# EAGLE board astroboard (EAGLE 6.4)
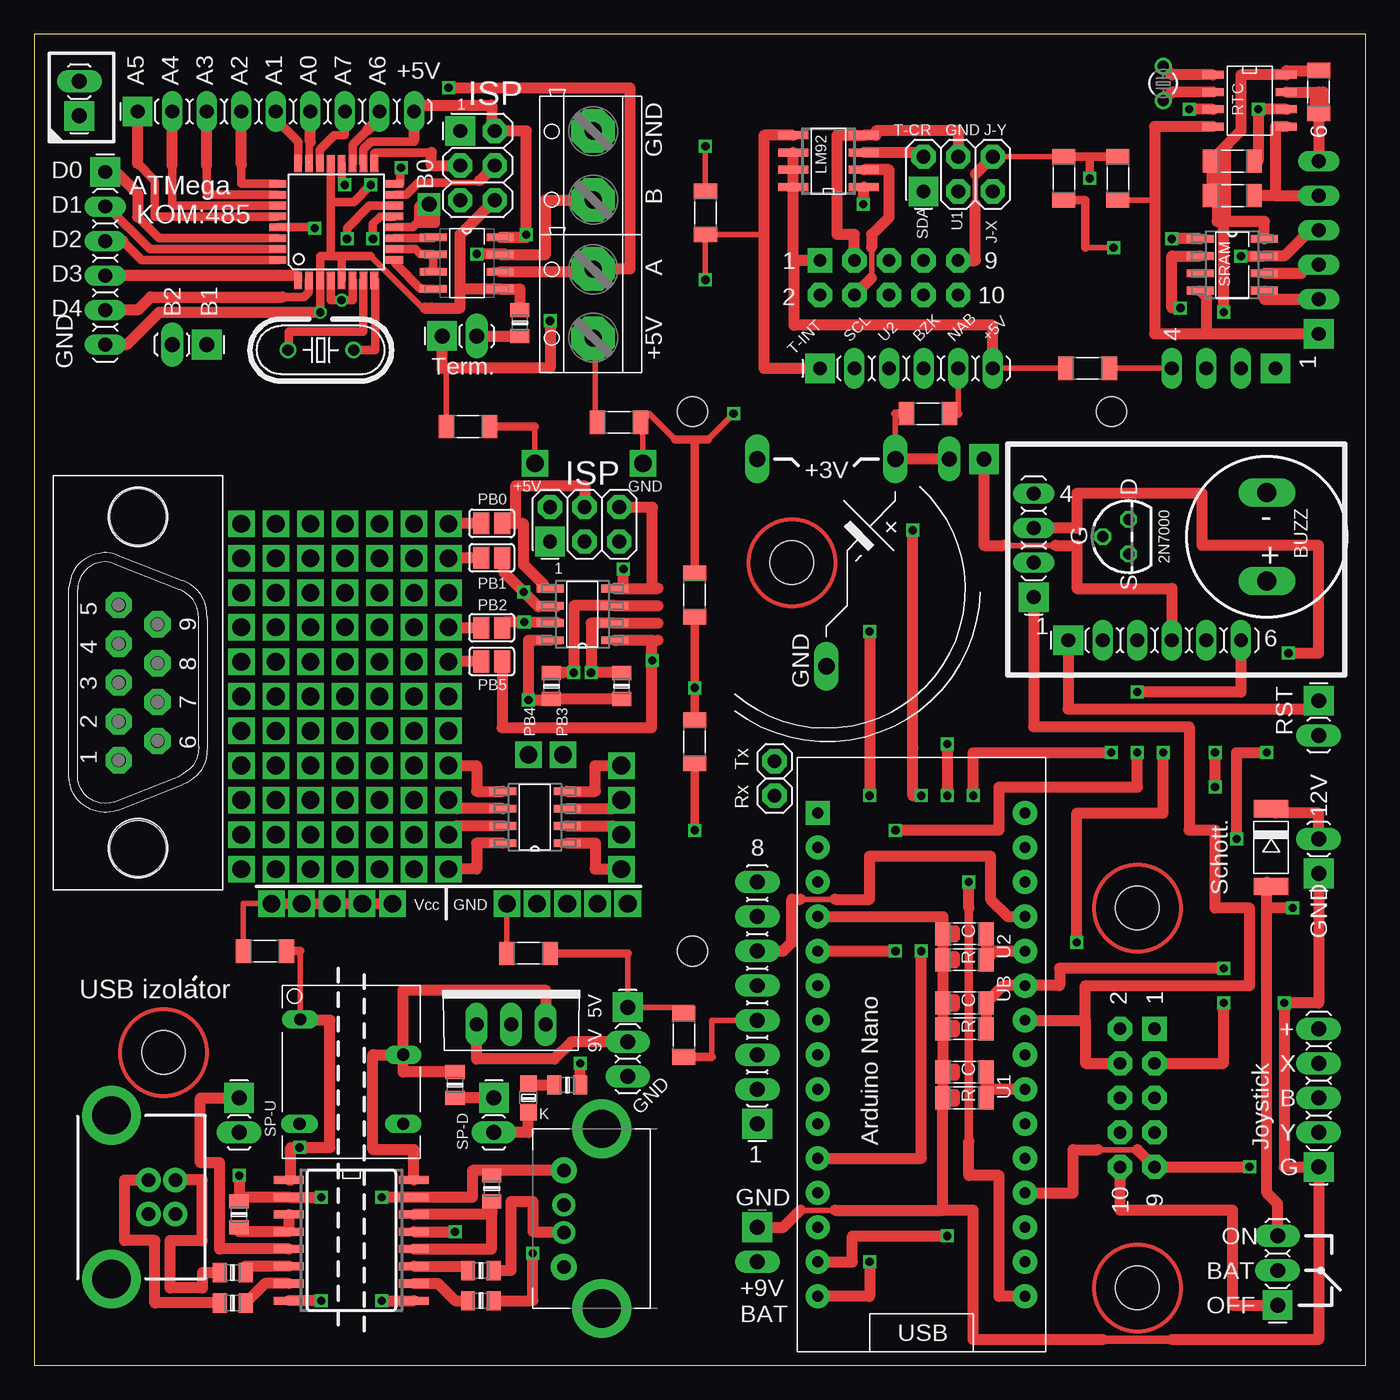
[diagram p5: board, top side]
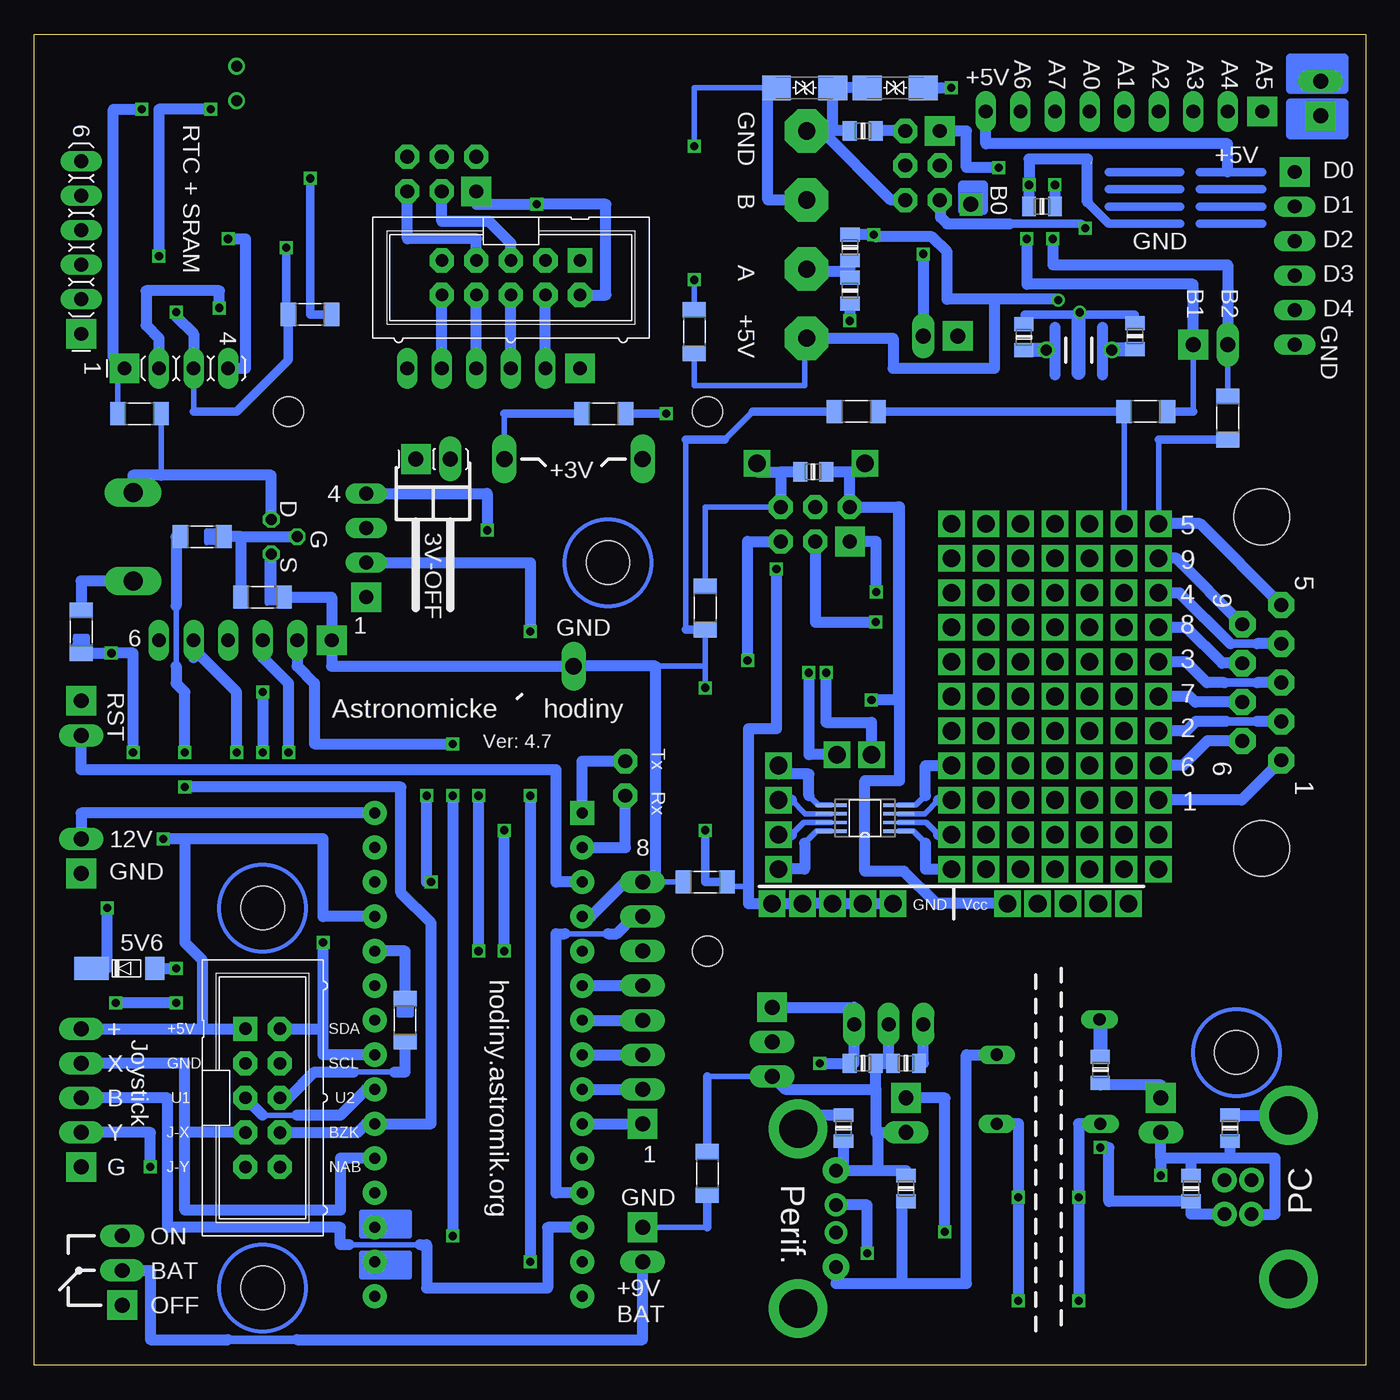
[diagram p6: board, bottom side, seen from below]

Size 97.93 x 97.94 mm. Coordinates in mm from the lower left corner, seen from the top.
Outline: 0,0 97.93,0 97.93,97.94 0,97.94 0,0
Copper layers (1*16): Top 0.0356mm / dielectric 1.5011mm / Bottom 0.0356mm
Design rules "LaenPCBOrder *": minimum track width 6mil, minimum drill 13mil, track to track 6mil, track to pad 6mil, pad to pad 6mil, via to via 6mil, smd to smd 6mil, copper to edge 15mil, drill to drill 6mil, minimum pad ring 7mil, minimum via ring 7mil, stop-mask expansion 3mil, vias tented up to drill 0mil, thermal gap 10mil
Holes 3.2 mm at 81.12,5.71 81.12,33.66 55.72,59.05 9.53,23.02
Holes 2.2 mm at 48.42,70.17 48.42,30.48 79.22,70.17

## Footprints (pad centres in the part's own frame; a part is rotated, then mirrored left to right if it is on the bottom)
BATTERY = drill 1.2 long: + 9.525,-5.08; +@1 9.525,5.08; - -5.715,0
BUZZER-12MM-NS = drill 1.4 long: + 3.25,0; - -3.25,0
1206 = smd 1.143 x 1.702: 1 -1.587,0; 2 1.587,0
0805 = smd 1.016 x 1.422: 1 -0.953,0; 2 0.953,0
CAN9V = drill 1.016 pad 1.93 octagon: 1 -5.715,0; 2 -2.857,0; 3 0,0; 4 2.857,0; 5 5.715,0; 6 -4.286,-2.857; 7 -1.429,-2.857; 8 1.429,-2.857; 9 4.286,-2.857 | hole 4.115: 12.192,-1.429; -12.192,-1.429
SM-1 = smd 1.27 x 2.54: A 2.857,0; K -2.857,0
SOD-80 = smd 1.397 x 1.702: A 1.905,0 | smd 2.54 x 1.702: K -2.731,0
SIM1-0505 = drill 0.9 long: 1 -3.756,3.867; 4 -3.81,-3.81; 5 3.81,-3.81; 7 3.81,1.27
SOIC127P600X175-8N = smd 1.981 x 0.559: 1 -2.362,1.905; 2 -2.362,0.635; 3 -2.362,-0.635; 4 -2.362,-1.905; 5 2.362,-1.905; 6 2.362,-0.635; 7 2.362,0.635; 8 2.362,1.905
TSSOP8 = smd 2.286 x 0.254: 1 -2.489,1.016; 2 -2.489,0.381; 3 -2.489,-0.254; 4 -2.489,-0.889; 5 2.489,-0.889; 6 2.489,-0.254; 7 2.489,0.381; 8 2.489,1.016
TO-220S = drill 1.016 pad 1.6 long: 1 -2.54,0; 2 0,0; 3 2.54,0
1X02 = drill 1.1 pad 2.184 square: 1 -1.27,0 | drill 1.1 long: 2 1.27,0
1X03 = drill 1.1 pad 2.184 square: 1 -2.54,0 | drill 1.1 long: 2 0,0; 3 2.54,0
2X03 = drill 1.016 pad 2.184 square: 1 -2.54,-1.27 | drill 1.016 pad 1.778 octagon: 2 -2.54,1.27; 3 0,-1.27; 4 0,1.27; 5 2.54,-1.27; 6 2.54,1.27
1X06 = drill 1.016 pad 2.184 square: 1 -6.35,0 | drill 1.016 long: 2 -3.81,0; 3 -1.27,0; 4 1.27,0; 5 3.81,0; 6 6.35,0
1X09 = drill 1.016 pad 2.184 square: 1 -10.16,0 | drill 1.016 long: 2 -7.62,0; 3 -5.08,0; 4 -2.54,0; 5 0,0; 6 2.54,0; 7 5.08,0; 8 7.62,0; 9 10.16,0
1X01 = drill 1.3 square: 1 0,0
1X08 = drill 1.1 pad 2.184 square: 1 -8.89,0 | drill 1.1 long: 2 -6.35,0; 3 -3.81,0; 4 -1.27,0; 5 1.27,0; 6 3.81,0; 7 6.35,0; 8 8.89,0
1X05 = drill 1.1 pad 2.184 square: 1 -5.08,0 | drill 1.1 long: 2 -2.54,0; 3 0,0; 4 2.54,0; 5 5.08,0
1X04 = drill 1.016 pad 2.184 square: 1 -3.81,0 | drill 1.016 long: 2 -1.27,0; 3 1.27,0; 4 3.81,0
MLW10G = drill 0.914 pad 1.778 square: 1 -5.08,-1.27 | drill 0.914 pad 1.778 octagon: 2 -5.08,1.27; 3 -2.54,-1.27; 4 -2.54,1.27; 5 0,-1.27; 6 0,1.27; 7 2.54,-1.27; 8 2.54,1.27; 9 5.08,-1.27; 10 5.08,1.27
1X02_OVAL = drill 1.1 pad 2.184 square: 1 -1.27,0 | drill 1.1 long: 2 1.27,0
1X01' = drill 1.016 pad 1.778 octagon: 1 0,0
ARK500/2 = drill 1.27 pad 3.2 octagon: 1 -2.54,0; 2 2.54,0
CHIP-LED0805 = smd 1.2 x 1.2: A 0,-1.05; C 0,1.05
PDIP-32 = drill 0.8 pad 1.778: 3V3 15.24,-35.56; +5V 15.24,-10.16; A0 15.24,-30.48; A1 15.24,-27.94; A2 15.24,-25.4; A3 15.24,-22.86; A4 15.24,-20.32; A5 15.24,-17.78; A6 15.24,-15.24; A7 15.24,-12.7; AREF 15.24,-33.02; D0/RX 0,-5.08; D2 0,-12.7; D3 0,-15.24; D4 0,-17.78; D5 0,-20.32; D6 0,-22.86; D7 0,-25.4; D8 0,-27.94; D9 0,-30.48; D10 0,-33.02; D11 0,-35.56; D12 0,-38.1; D13 15.24,-38.1; GND 0,-10.16; GND1 15.24,-5.08; RESET 0,-7.62; RESET1 15.24,-7.62; VIN 15.24,-2.54 | drill 0.8 pad 1.778 square: D1/TX 0,-2.54
TQFP32-08 = smd 1.27 x 0.559: 1 -4.293,2.8; 2 -4.293,2; 3 -4.293,1.2; 4 -4.293,0.4; 5 -4.293,-0.4; 6 -4.293,-1.2; 7 -4.293,-2; 8 -4.293,-2.8; 17 4.293,-2.8; 18 4.293,-2; 19 4.293,-1.2; 20 4.293,-0.4; 21 4.293,0.4; 22 4.293,1.2; 23 4.293,2; 24 4.293,2.8 | smd 0.559 x 1.27: 9 -2.8,-4.293; 10 -2,-4.293; 11 -1.2,-4.293; 12 -0.4,-4.293; 13 0.4,-4.293; 14 1.2,-4.293; 15 2,-4.293; 16 2.8,-4.293; 25 2.8,4.293; 26 2,4.293; 27 1.2,4.293; 28 0.4,4.293; 29 -0.4,4.293; 30 -1.2,4.293; 31 -2,4.293; 32 -2.8,4.293
TC26V = drill 0.813: 1 -1.27,0; 2 1.27,0
HC49U-V = drill 0.813: 1 -2.413,0; 2 2.413,0
SJ-NC = smd 1.168 x 1.6: 1 -0.762,0; 2 0.762,0
TO-92 = drill 0.813 octagon: 1 -1.27,0; 2 1.27,0; 3 0,1.905
DO214AC+MINIMELF_BIDIR = smd 2.123 x 1.8: P$1 -2.064,0; P$2 2.064,0
SO-8 = smd 0.6 x 1.55: 1 -1.905,-2.69; 2 -0.635,-2.69; 3 0.635,-2.69; 4 1.905,-2.69; 5 1.905,2.71; 6 0.635,2.71; 7 -0.635,2.71; 8 -1.905,2.71
SO08 = smd 0.6 x 2.2: 1 -1.905,-2.6; 2 -0.635,-2.6; 3 0.635,-2.6; 4 1.905,-2.6; 5 1.905,2.6; 6 0.635,2.6; 7 -0.635,2.6; 8 -1.905,2.6
SO16W = smd 0.6 x 2.2: 1 -4.445,-4.6; 2 -3.175,-4.6; 3 -1.905,-4.6; 4 -0.635,-4.6; 5 0.635,-4.6; 6 1.905,-4.6; 7 3.175,-4.6; 8 4.445,-4.6; 9 4.445,4.6; 10 3.175,4.6; 11 1.905,4.6; 12 0.635,4.6; 13 -0.635,4.6; 14 -1.905,4.6; 15 -3.175,4.6; 16 -4.445,4.6
SOIC127P600X175-8N' = smd 1.981 x 0.559: 1 -2.464,1.905; 2 -2.464,0.635; 3 -2.464,-0.635; 4 -2.464,-1.905; 5 2.464,-1.905; 6 2.464,-0.635; 7 2.464,0.635; 8 2.464,1.905
USB-B-PTH = drill 1 pad 1.778: D+ 0,1.25; D- 1.981,1.25; GND 0,-1.25; VBUS 1.981,-1.25 | drill 2.8 pad 4.318: P$2 -2.718,6.02; SHIELD -2.718,-6.02
USB-A-H = drill 1 pad 1.676: D+ 2.794,-1.016; D- 2.794,1.016 | drill 1 pad 1.93: GND 2.794,-3.556; VBUS 2.794,3.556 | drill 2.8 pad 4.318: SHIELD@1 0,-6.604; SHIELD@2 0,6.604

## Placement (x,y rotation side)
BAT3V  3V  [BATTERY]  58.26,57.15 90 top
BUZZ  LD-BZEN1205  [BUZZER-12MM-NS]  90.65,60.96 270 top
C1  100n  [1206]  68.42,24.77 0 top
C2  100n  [1206]  68.42,29.84 0 top
C3  100n  [1206]  68.42,19.68 0 top
C4  100n  [0805]  12.86,13.02 90 bottom
C5  100n  [0805]  15.08,11.11 90 top
C6  100n  [0805]  10,17.46 270 bottom
C7  100n  [0805]  33.81,13.02 90 bottom
C8  100n  [0805]  33.66,13.02 90 top
C9  100n  [0805]  38.42,17.46 90 bottom
C10  100n  [0805]  36.99,22.23 0 bottom
C11  100n  [0805]  33.81,22.23 180 bottom
C12  1u  [0805]  23.81,85.25 180 bottom
C13  18p  [0805]  16.98,75.71 90 bottom
C14  18p  [0805]  25.15,75.63 90 bottom
C15  1uF  [0805]  36.99,90.81 0 bottom
C16  1uF  [0805]  40.64,65.72 180 bottom
CAN1  CAN_9V  [CAN9V]  6.22,50.23 90 top
D1  SK110  [SM-1]  90.96,38.1 270 top
D2  5V6  [SOD-80]  90.96,29.21 0 bottom
DC-DC1  [SIM1-0505]  23.34,21.59 0 top
EMPTY1  SOIC-NIC  [SOIC127P600X175-8N]  36.83,40.32 180 top
EMPTY2  TSSOP-NIC  [TSSOP8]  36.83,40.32 180 bottom
IO1  7805  [TO-220S]  35.08,25.08 0 top
JP1  [1X02]  15.08,18.41 270 top
JP2  [1X02]  33.81,18.41 270 top
JP3  [1X03]  43.66,23.81 270 top
JP4  [1X02]  31.27,75.72 0 top
JP5  [2X03]  32.61,88.26 270 top
JP6  [1X06]  5.24,81.44 270 top
JP7  [1X02]  11.43,75.09 180 top
JP8  [1X09]  17.78,92.23 0 top
JP9  [1X02]  3.33,93.19 90 top
JP10  [2X03]  40.48,61.88 0 top
JP11  [1X01]  30.48,39.05 0 top
JP12  [1X01]  30.48,41.59 0 top
JP13  [1X01]  30.48,44.13 0 top
JP14  [1X01]  43.18,36.51 180 top
JP15  [1X01]  43.18,39.05 180 top
JP16  [1X01]  43.18,41.59 180 top
JP17  [1X01]  43.18,44.13 180 top
JP18  [1X01]  15.24,41.59 0 top
JP19  [1X01]  15.24,46.67 180 top
JP20  [1X01]  15.24,51.75 180 top
JP21  [1X01]  15.24,56.83 180 top
JP22  [1X01]  15.24,61.91 180 top
JP23  [1X01]  15.24,44.13 180 top
JP24  [1X01]  15.24,49.21 180 top
JP25  [1X01]  15.24,54.29 180 top
JP26  [1X01]  15.24,59.37 180 top
JP27  [1X01]  30.48,61.91 90 top
JP28  [1X01]  30.48,59.37 90 top
JP29  [1X01]  30.48,54.29 90 top
JP30  [1X01]  30.48,51.75 90 top
JP31  [1X01]  38.89,44.93 90 top
JP32  [1X01]  36.35,44.93 90 top
JP33  [1X01]  22.86,39.05 0 top
JP34  [1X01]  17.78,61.91 0 top
JP35  [1X01]  20.32,61.91 0 top
JP36  [1X01]  22.86,61.91 0 top
JP37  [1X01]  17.78,59.37 0 top
JP38  [1X01]  25.4,61.91 0 top
JP39  [1X01]  27.94,61.91 0 top
JP40  [1X01]  20.32,59.37 0 top
JP41  [1X01]  25.4,59.37 0 top
JP42  [1X01]  22.86,59.37 0 top
JP43  [1X01]  17.78,56.83 0 top
JP44  [1X01]  27.94,59.37 0 top
JP45  [1X01]  20.32,56.83 0 top
JP46  [1X01]  22.86,56.83 0 top
JP47  [1X01]  25.4,56.83 0 top
JP48  [1X01]  27.94,56.83 0 top
JP49  [1X01]  17.78,54.29 0 top
JP50  [1X01]  30.48,56.83 0 top
JP51  [1X01]  25.4,41.59 0 top
JP52  [1X01]  22.86,51.75 0 top
JP53  [1X01]  20.32,54.29 0 top
JP54  [1X01]  22.86,46.67 0 top
JP55  [1X01]  27.94,49.21 0 top
JP56  [1X01]  25.4,54.29 0 top
JP57  [1X01]  20.32,46.67 0 top
JP58  [1X01]  30.48,49.21 0 top
JP59  [1X01]  27.94,54.29 0 top
JP60  [1X01]  22.86,54.29 0 top
JP61  [1X01]  17.78,46.67 0 top
JP62  [1X01]  30.48,46.67 0 top
JP63  [1X01]  25.4,51.75 0 top
JP64  [1X01]  17.78,51.75 0 top
JP65  [1X01]  17.78,44.13 0 top
JP66  [1X01]  27.94,46.67 0 top
JP67  [1X01]  20.32,49.21 0 top
JP68  [1X01]  17.78,49.21 0 top
JP69  [1X01]  25.4,39.05 0 top
JP70  [1X01]  25.4,46.67 0 top
JP71  [1X01]  22.86,49.21 0 top
JP72  [1X01]  20.32,51.75 0 top
JP73  [1X01]  20.32,44.13 0 top
JP74  [1X01]  25.4,44.13 0 top
JP75  [1X01]  25.4,49.21 0 top
JP76  [1X01]  27.94,51.75 0 top
JP77  [1X01]  22.86,41.59 0 top
JP78  [1X01]  20.32,41.59 0 top
JP79  [1X01]  17.78,41.59 0 top
JP80  [1X01]  22.86,44.13 0 top
JP81  [1X01]  15.24,36.51 0 top
JP82  [1X01]  20.32,39.05 0 top
JP83  [1X01]  17.78,36.51 0 top
JP84  [1X01]  17.78,39.05 0 top
JP85  [1X01]  20.32,36.51 0 top
JP86  [1X01]  15.24,39.05 0 top
JP87  [1X01]  25.4,36.51 0 top
JP88  [1X01]  22.86,36.51 0 top
JP89  [1X01]  27.94,44.13 0 top
JP90  [1X01]  27.94,41.59 0 top
JP91  [1X01]  27.94,39.05 0 top
JP92  [1X01]  27.94,36.51 0 top
JP93  [1X01]  34.77,33.97 0 top
JP94  [1X01]  44.77,66.36 0 top
JP95  [1X01]  36.83,66.36 0 top
JP97  [1X01]  36.99,33.97 0 top
JP98  [1X01]  39.21,33.97 0 top
JP99  [1X01]  41.43,33.97 0 top
JP100  [1X01]  43.66,33.97 0 top
JP101  [1X01]  19.68,33.97 0 top
JP103  [1X01]  21.91,33.97 0 top
JP104  [1X01]  17.46,33.97 0 top
JP105  [1X01]  26.35,33.97 0 top
JP106  [1X01]  24.13,33.97 0 top
JP108  [1X01]  30.48,36.51 0 top
K1  [1X08]  53.18,26.67 90 top
K2  [1X05]  94.46,19.68 90 top
K3A  [1X04]  73.5,60.33 90 top
K3B  [1X04]  87.47,73.34 180 top
K4A  [1X06]  82.39,53.34 0 top
K4B  [1X06]  94.46,82.23 90 top
K5  MLW10  [MLW10G]  81.12,19.68 270 bottom
K6  [1X02]  94.46,37.47 90 top
K7  [1X02_OVAL]  53.18,8.89 270 top
K8  [1X03]  91.44,6.99 90 top
K9  [1X02]  94.46,47.62 270 top
K10  [1X01']  54.45,44.45 0 top
K11  [1X01']  54.45,41.91 0 top
K12  [1X02]  68.58,66.67 0 bottom
K13  MLW10  [MLW10G]  62.87,80.01 180 bottom
K14  [2X03]  67.94,87.63 0 top
K15  [1X06]  64.14,73.34 0 top
K16A  ARK500/2  [ARK500/2]  41.12,78.11 90 top
K16B  ARK500/2  [ARK500/2]  41.12,88.27 90 top
LED1  [CHIP-LED0805]  36.35,19.68 180 top
MCU1  ARDUINONANO  [PDIP-32]  57.63,43.18 0 top
MCU2  ATTINY__  [SOIC127P600X175-8N]  40.32,55.24 180 top
MCU3  ATmega328  [TQFP32-08]  22.22,84.11 90 top
Q1  32768Hz  [TC26V]  83.03,94.3 90 top
Q2  16MHz  [HC49U-V]  21.09,74.69 180 top
R1  4k7  [1206]  85.57,60.96 0 bottom
R2  18k  [1206]  81.12,56.52 180 bottom
R3  330R  [1206]  94.46,53.98 90 bottom
R4  3k3  [1206]  94.46,93.66 90 top
R5  3k3  [1206]  88.11,88.58 180 top
R6  3k3  [1206]  88.11,86.04 180 top
R7  10k  [1206]  68.42,26.67 0 top
R8  1k  [1206]  75.72,87.31 90 top
R8-A  0R  [1206]  70.64,25.4 270 bottom
R8-B  10k  [1206]  68.42,31.75 0 top
R9  10k  [1206]  68.42,21.59 0 top
R10  24R 1%  [0805]  14.61,6.83 0 top
R11  24R 1%  [0805]  14.61,4.6 0 top
R12  47k  [0805]  19.53,21.75 90 bottom
R13  24R 1%  [0805]  32.86,6.99 0 top
R14  24R 1%  [0805]  32.86,4.76 0 top
R15  47k  [0805]  30.96,20.64 90 top
R16  1k  [0805]  39.21,20.64 0 top
R17  47k  [0805]  35.72,76.68 90 top
R18  47k  [0805]  37.94,82.23 270 bottom
R19  120R  [0805]  37.94,79.06 90 bottom
R20  47k  [0805]  43.21,49.97 270 top
R21  47k  [0805]  38.04,49.97 270 top
R22  1k  [1206]  79.69,87.31 270 top
R23  1k  [1206]  90.17,70.01 180 bottom
R24  1k  [1206]  65.72,70.01 0 top
R25  1k  [1206]  77.47,73.34 180 top
R26  1k  [1206]  49.37,84.77 90 top
R27  1k  [1206]  48.58,35.56 0 bottom
R28  1k  [1206]  48.58,55.72 90 bottom
R29  1k  [1206]  48.58,45.88 270 top
R30  1k  [1206]  10.16,69.69 270 bottom
R31  1k  [1206]  49.37,76.04 270 bottom
R32  1k  [1206]  16.19,70.17 180 bottom
R33  1k  [1206]  77.63,77.31 180 bottom
R34  1k  [1206]  31.91,69.06 0 top
R35  1k  [1206]  43.02,69.37 180 top
R36  1k  [1206]  47.78,24.29 270 top
R37  1k  [1206]  48.42,14.13 270 bottom
R38  1k  [1206]  16.99,30.48 0 top
R39  1k  [1206]  36.35,30.32 0 top
R40  1k  [1206]  37.47,70.17 0 bottom
R41  1k  [1206]  48.58,56.67 270 top
R42  1k  [1206]  56.04,70.01 180 bottom
SJ-B0  SOLDERJUMPERNC  [SJ-NC]  33.66,61.94 180 top
SJ-B1  SOLDERJUMPERNC  [SJ-NC]  33.66,59.4 180 top
SJ-B2  SOLDERJUMPERNC  [SJ-NC]  33.66,54.26 180 top
SJ-B5  SOLDERJUMPERNC  [SJ-NC]  33.66,51.78 180 top
T1  2N7000  [TO-92]  80.49,60.96 90 top
TR1  6V8  [DO214AC+MINIMELF_BIDIR]  41.27,93.98 180 bottom
TR2  6V8  [DO214AC+MINIMELF_BIDIR]  34.61,93.98 0 bottom
U1  23LCV512-I/SN  [SOIC127P600X175-8N]  88.11,80.96 0 top
U2  RTC-M41T81M6F  [SO-8]  89.38,93.03 270 top
U3  LM92  [SO08]  58.42,88.58 90 top
U4  ADuM4160  [SO16W]  23.34,9.21 270 top
U5  ADM485ARZ  [SOIC127P600X175-8N']  31.83,81.08 0 top
X1  USB B  [USB-B-PTH]  8.41,12.38 0 top
X2  USB A  [USB-A-H]  41.75,10.79 180 top

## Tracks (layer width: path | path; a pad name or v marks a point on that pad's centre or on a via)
+3V(BAT)
  Top 0.406: 71.28,60.33 75.09,60.33
  Top 0.813: K4A.4 83.66,57.15 76.68,57.15 76.68,60.33 75.09,60.33 | 71.28,60.33 69.85,60.33 K12.1
+3V(BAT)-ED  (via drill 0.6)
  Top 0.813: U2.3 v84.93,92.39 | v88.74,81.6 U1.7 91.92,81.6 93.82,83.5 K4B.4
  Bottom 0.813: v84.93,92.39 88.74,92.39 v88.74,81.6
+5V  (via drill 0.6)
  Top 0.406: 56.36,34.29 58.9,34.29
  Top 0.813: K1.6 55.09,30.48 55.72,31.11 55.72,34.29 56.36,34.29 | MCU1.+5V 71.6,33.02 70.33,34.29 70.33,37.47 61.44,37.47 61.44,34.29 58.9,34.29 | v92.23,52.39 R3.1 94.46,60.33 85.88,60.33 85.88,64.14 76.68,64.14 76.68,61.59 K3A.3 | v88.42,38.73 88.42,45.09 v90.65,45.09
  Bottom 0.305: 94.93,52.86 94.93,53.18 | 94.93,53.5 94.93,53.66 93.98,53.66 93.98,53.5 | 94.93,53.34 94.93,53.18 | 94.93,53.18 94.14,53.18 | 93.98,53.5 93.98,53.34 | 93.98,53.34 93.98,53.02 | 93.98,53.34 94.93,53.34 | 94.93,53.34 94.93,53.5 | 94.93,53.5 93.98,53.5
  Bottom 0.406: 93.82,52.86 94.46,52.86 | 94.46,52.86 94.93,52.86 95.09,52.86 | R3.1 94.46,52.86
  Bottom 0.813: K2.5 85.57,24.77 | 85.57,24.77 K5.1 | MCU1.+5V 76.68,33.02 76.68,38.73 86.84,38.73 | 86.84,38.73 86.84,31.11 85.57,29.84 85.57,24.77 | 86.84,38.73 v88.42,38.73 | v90.65,45.09 90.65,52.39 v92.23,52.39 R3.1
+5V-ED  (via drill 0.6)
  Top 0.406: 87.47,84.14 87.47,84.45 | v79.38,82.23 77.31,82.23
  Top 0.61: U2.8 92.09,95.25 | R6.2 R5.2 87,89.06 | R8.1 77.31,85.72 77.31,82.23
  Top 0.813: 92.09,95.25 R4.2 | U2.8 88.74,94.93 88.74,90.81 87,89.06 87,84.14 87.47,84.14 | U1.8 90.47,84.14 87.47,84.14 | v87.47,77.47 87.47,84.14
  Top 1.016: 87.47,89.38 87.47,84.45
  Bottom 0.406: R33.2 79.38,77.31 79.38,73.66 | 86.2,70.17 K3B.3
  Bottom 0.61: 79.38,77.31 v79.38,82.23 | 86.2,70.17 83.03,70.17 79.22,73.98 R33.2
  Bottom 0.813: v87.47,77.47 87.47,77.15 86.2,75.88 K3B.3
+5V-TP
  Top 0.406: R25.2 K15.6
  Top 0.813: K13.1 55.88,81.28 | 55.88,81.28 55.82,81.28 U3.8 U3.7 U3.6 | K15.6 70.48,76.52 55.88,76.52 55.88,81.28
ARDU/3V3
  Bottom 0.406: MCU1.3V3 70.33,7.62 | 70.33,7.62 70.33,7.3 | 70.33,7.3 70.33,6.51 73.82,6.51 73.82,8.26 70.33,8.26 70.33,7.62 | 70.33,7.3 70.64,7.3 | 70.64,6.99 70.64,6.67 73.5,6.67 73.5,7.3 70.64,7.3 | 70.64,7.3 70.64,7.94 73.18,7.94 73.18,7.62 | 70.64,7.3 70.64,6.99 | 70.64,6.99 73.34,6.99 73.34,7.46 72.55,7.46
  Bottom 0.61: 73.18,7.62 73.18,7.3
ARDU/A0  (via drill 0.6)
  Top 0.406: 78.23,15.88 81.12,15.88
  Top 0.813: v89.38,14.61 K5.9 81.12,15.88 | MCU1.A0 76.4,12.7 76.4,15.88 78.23,15.88
  Bottom 0.813: v89.38,14.61 89.38,17.14 K2.2
ARDU/A0-TP  (via drill 0.6)
  Top 0.406: 69.22,85.41 69.22,87.63 | K14.6 R8.2
  Top 0.61: R8.2 77.63,88.9 | 77.63,88.9 R22.1 | v77.63,87.31 77.63,88.9
  Top 0.813: K13.9 69.22,81.28 69.22,85.41 | 69.22,87.63 K14.6
  Bottom 0.61: R33.1 77.63,77.31 v77.63,87.31
ARDU/A1
  Bottom 0.813: MCU1.A1 75.41,15.24 75.41,11.43 86.84,11.43 86.84,17.14 | 86.84,17.14 86.84,22.23 K2.4 | K5.7 86.84,17.14
ARDU/A1-TP
  Bottom 0.813: K13.7 65.41,82.87 70.48,82.87 K14.5
ARDU/A2  (via drill 0.6)
  Top 0.813: v86.84,42.55 v86.84,45.09
  Bottom 0.406: 87.47,55.88 87.47,51.44
  Bottom 0.813: v86.84,42.55 70.96,42.55 70.96,34.77 68.74,32.54 68.74,17.78 MCU1.A2 73.5,17.78 74.14,17.14 K5.8 | v86.84,45.09 86.84,49.53 87.47,50.16 87.47,51.44 | R1.1 87.47,60.96 87.47,55.88
ARDU/A2-TP
  Bottom 0.813: K15.4 K13.8
ARDU/A3
  Top 0.61: C3.2 70.01,20.32
  Top 0.813: R9.2 70.01,20.32 MCU1.A3
  Bottom 0.406: 78.58,18.41 81.12,18.41
  Bottom 0.813: K5.5 81.12,18.41 | MCU1.A3 73.5,20.32 75.41,18.41 78.58,18.41
ARDU/A3-TP
  Bottom 0.813: K13.5 62.87,82.55 64.45,84.14 67.94,84.14 K14.3
ARDU/A4  (via drill 0.6)
  Top 0.813: v76.68,31.11 76.68,40.64 83.03,40.64 v83.03,45.09
  Bottom 0.813: MCU1.A4 76.68,22.86 76.68,24.77 | K5.2 76.68,24.77 | 76.68,24.77 v76.68,31.11 | v83.03,45.09 83.03,49.53 86.2,52.7 | 86.2,52.07 86.2,52.7 | 86.2,52.7 K4A.5
ARDU/A4-ED
  Top 0.813: U2.5 91.28,91.12 91.28,86.04 | 91.28,86.04 R6.1 | 91.28,86.04 K4B.5
ARDU/A4-TP  (via drill 0.6)
  Top 0.406: v60.96,85.41 61.02,85.41
  Top 0.813: 61.02,85.41 U3.1
  Bottom 0.813: K13.2 55.88,78.74 55.88,85.41 v60.96,85.41 65.41,85.41 K14.1
ARDU/A5
  Top 0.813: MCU1.A5 77.31,25.4 | 77.31,25.4 77.31,22.23 K5.4 | K3A.1 73.5,46.99 84.93,46.99 84.93,39.37 86.84,39.37 86.84,33.66 89.38,33.66 89.38,27.94 77.31,27.94 77.31,25.4
ARDU/A5-ED  (via drill 0.6)
  Top 0.61: 90.01,88.58 R5.1
  Top 0.813: U2.6 v90.01,92.39 90.01,88.58
  Bottom 0.406: K3B.1 91.76,73.34 R23.2
  Bottom 0.813: K3B.1 92.09,74.15 U2.6 v90.01,92.39
ARDU/A5-TP
  Top 0.406: 61.59,82.23 61.59,80.01
  Top 0.813: K13.4 61.59,80.01 | U3.2 62.87,87.95 62.87,84.45 61.59,83.19 61.59,82.23
  Bottom 0.813: K15.2 K13.4
ARDU/A6  (via drill 0.6)
  Top 0.813: C1.2 R7.2 71.28,27.94 MCU1.A6 75.41,27.94 75.41,29.21 v87.47,29.21
  Bottom 0.813: D2.A v87.47,29.21
ARDU/A7
  Top 0.813: R8-B.2 C2.2 70.64,30.48 MCU1.A7
  Bottom 0.305: 70.17,26.51 70.17,25.72 71.12,25.72 71.12,26.51 70.33,26.51 70.33,25.88 70.96,25.88 70.96,26.35 70.48,26.35 70.48,26.04 | 70.8,26.04 70.8,26.19
  Bottom 0.406: 70.48,26.04 70.8,26.04 | 70.33,26.51 70.64,26.51 R8-A.1
  Bottom 0.813: R8-A.1 70.64,30.48 MCU1.A7
ARDU/A7-TP
  Bottom 0.813: K15.3 K13.6
ARDU/AREF
  Bottom 0.406: MCU1.AREF 70.33,10.16 | 70.33,10.16 70.33,9.84 | 70.33,9.84 70.33,9.53 73.82,9.53 73.82,11.27 70.33,11.27 70.33,10.64 | 70.33,10.16 70.33,10.48 70.33,10.64 | 70.33,9.84 73.5,9.84 73.5,10 | 73.5,10.64 73.5,10.95 70.64,10.95 70.64,10.48 73.18,10.48 73.18,10 73.5,10 | 73.5,10 73.5,10.64 | 73.5,10.64 70.33,10.64
ARDU/D0
  Bottom 0.813: MCU1.D0/RX 54.45,38.1 K11.1
ARDU/D1
  Bottom 0.813: MCU1.D1/TX 57.63,44.45 K10.1
ARDU/D2  (via drill 0.6)
  Top 0.813: MCU1.D2 v63.34,30.48 | K4A.6 88.74,49.53 v81.12,49.53 | v63.34,39.37 70.96,39.37 70.96,42.55 81.12,42.55 v81.12,45.09
  Bottom 0.813: v81.12,49.53 v81.12,45.09 | v63.34,30.48 v63.34,39.37
ARDU/D2-ED
  Top 0.406: 93.98,92.71 94.93,92.71 94.93,93.66 | 93.98,93.03 94.93,93.03 | 93.98,93.03 93.98,93.5 | 94.93,93.66 94.93,93.82 | 94.77,93.66 94.93,93.66 | 93.98,92.55 93.98,92.71 | 93.98,93.03 93.98,92.87 93.98,92.71
  Top 0.813: U2.7 94.46,93.66 | 94.46,93.66 R4.1 K4B.6 | 94.46,93.66 94.77,93.66 94.77,92.55
ARDU/D3
  Bottom 0.813: MCU1.D3 K1.5
ARDU/D4
  Top 0.406: 49.85,22.7 49.85,25.4 K1.4
  Top 0.61: R36.2 49.85,22.7
  Bottom 0.813: MCU1.D4 K1.4
ARDU/D5
  Bottom 0.813: MCU1.D5 K1.3
ARDU/D6
  Bottom 0.813: MCU1.D6 K1.2
ARDU/D7
  Bottom 0.813: MCU1.D7 K1.1
ARDU/D8  (via drill 0.6)
  Top 0.813: MCU1.D8 65.25,15.24 v65.25,30.48 | v65.25,41.91 64.61,41.91 64.61,45.4 v64.61,61.44
  Bottom 0.813: v65.25,30.48 v65.25,41.91 | K3A.4 64.61,64.14 v64.61,61.44
ARDU/D8-ED  (via drill 0.6)
  Top 0.406: R25.1 K3B.4
  Top 0.813: U1.1 v83.66,82.87
  Bottom 0.813: v83.66,82.87 82.39,82.87 82.39,73.34 K3B.4
ARDU/D9
  Bottom 0.406: 58.9,31.75 55.72,31.75
  Bottom 0.813: MCU1.D9 59.53,12.7 59.53,31.75 58.9,31.75 | 55.72,31.75 55.09,31.75 53.82,33.02 K1.7
ARDU/D10
  Bottom 0.406: 69.53,8.89 74.77,8.89
  Bottom 0.813: K2.3 88.11,19.68 88.11,10.16 75.41,10.16 75.41,8.89 74.77,8.89 | MCU1.D10 60.17,10.16 60.17,5.71 69.06,5.71 69.06,8.89 69.53,8.89
ARDU/D11  (via drill 0.6)
  Top 0.813: v67.15,45.72 v67.15,41.91 | MCU1.D11 60.17,7.62 60.17,9.53 v67.15,9.53
  Bottom 0.813: K4A.2 78.58,51.44 77.31,50.16 77.31,45.72 v67.15,45.72 | v67.15,41.91 v67.15,9.53
ARDU/D11-ED
  Top 0.813: U1.5 90.47,78.42 K4B.2
ARDU/D12  (via drill 0.6)
  Top 0.813: v61.44,53.98 v61.44,41.91 | v61.44,7.62 61.44,5.08 MCU1.D12
  Bottom 0.813: K3A.2 61.44,59.05 v61.44,53.98 | v61.44,41.91 v61.44,7.62
ARDU/D12-ED  (via drill 0.6)
  Top 0.813: v84.3,77.79 83.66,77.79 83.66,81.6 U1.2
  Bottom 0.813: v84.3,77.79 84.3,79.06 89.69,79.06 89.69,76.52 88.74,75.56 K3B.2
ARDU/D13  (via drill 0.6)
  Top 0.61: 68.74,16.51 68.74,33.66
  Top 0.813: MCU1.D13 70.96,5.08 70.96,13.97 68.74,13.97 68.74,16.51 | v69.06,41.91 69.06,45.09 v79.22,45.09 | 68.74,33.66 v68.74,35.56
  Bottom 0.813: v68.74,35.56 69.06,35.56 v69.06,41.91 | v79.22,45.09 79.22,50.16 81.12,52.07 K4A.3
ARDU/D13-ED
  Top 0.813: U1.6 93.19,80.33 93.82,80.96 K4B.3
ARDU/RESET
  Bottom 0.813: MCU1.RESET 59.53,35.56 59.53,43.81 94.46,43.81 K9.2
ARDU/VIN
  Top 0.813: K6.2 94.46,40.64 91.28,40.64 D1.K
  Bottom 0.813: MCU1.VIN 94.46,40.64 K6.2
ARDUKOM/B0  (via drill 1.1)
  Top 0.61: 28.26,84.77 28.26,85.25 28.57,85.57 28.57,85.72 29.53,85.72 29.53,85.25 | 29.21,83.98 28.73,83.98 | 28.73,83.98 28.26,83.98 28.26,84.77 | 28.26,84.77 28.73,84.77 28.73,84.61 | 28.73,84.61 28.73,84.3 | MCU3.12 27.83,83.71 28.73,84.61 | 28.73,83.98 28.73,85.41 v29.05,85.41 29.21,85.41 29.21,85.25 | 29.21,85.25 29.21,83.98 | 29.21,83.98 29.53,83.98 29.53,85.25 | 29.53,85.25 29.21,85.25
  Bottom 0.61: 29.53,84.93 28.1,84.93 28.1,86.84 29.69,86.84 29.69,84.93 29.37,84.93 29.37,86.36 29.05,86.36 | 29.05,86.36 28.57,86.36 28.57,85.09 29.05,85.09 v29.05,85.41 29.05,86.36
ARDUKOM/B1  (via drill 0.6)
  Top 0.61: MCU3.13 25.45,84.51 24.92,83.98 v24.92,82.87
  Bottom 0.406: JP7.1 12.7,70.17
  Bottom 0.61: 12.7,70.17 R32.1
  Bottom 0.813: v24.92,82.87 24.92,79.53 12.7,79.53 JP7.1
ARDUKOM/B2  (via drill 0.6)
  Top 0.61: MCU3.14 24.67,85.31 23.02,83.66 v23.02,82.87
  Bottom 0.406: JP7.2 R30.1
  Bottom 0.813: v23.02,82.87 23.02,80.96 10.16,80.96 JP7.2
ARDUKOM/C0  (1 unrouted)
  Top 0.406: MCU3.23 20.32,88.4 20.32,90.01 | 20.16,88.58 20.16,90.17
  Top 0.813: 20.32,90.01 JP8.6
ARDUKOM/C1
  Top 0.61: MCU3.24 19.42,90.01 17.83,91.6 17.78,91.6
  Top 0.813: JP8.5 17.78,91.6
ARDUKOM/C2
  Top 0.406: 15.24,91.28 JP8.4
  Top 0.61: MCU3.25 15.24,86.91 15.24,88.34
  Top 0.813: 15.24,88.34 JP8.4
ARDUKOM/C3
  Top 0.61: MCU3.26 12.7,86.11 12.7,88.27
  Top 0.813: 12.7,88.27 JP8.3
ARDUKOM/C4
  Top 0.61: MCU3.27 10.16,85.31 10.16,88.27
  Top 0.813: 10.16,88.27 JP8.2
ARDUKOM/C5
  Top 0.61: MCU3.28 8.89,84.51 8.89,87.15 7.62,88.42
  Top 0.813: 7.62,88.42 JP8.1
ARDUKOM/C6
  Top 0.61: MCU3.19 23.42,89.78 24.53,90.88
  Top 0.813: JP8.8 25.4,91.76 24.53,90.88
ARDUKOM/C7
  Top 0.61: MCU3.22 21.02,89.44 22.07,90.49 22.86,90.49 JP8.7
ARDUKOM/D0
  Top 0.61: MCU3.30 9.21,82.91 7.62,84.5
  Top 0.813: 7.62,84.5 7.62,86.2 6.03,87.79 JP6.1
ARDUKOM/D1
  Top 0.61: MCU3.31 8.54,82.11 5.4,85.25
  Top 0.813: JP6.2 5.4,85.25
ARDUKOM/D2
  Top 0.61: MCU3.32 7.94,81.31 6.54,82.71
  Top 0.813: 6.54,82.71 JP6.3
ARDUKOM/D3
  Top 0.61: MCU3.1 19.42,80.17 19.21,80.17
  Top 0.813: 19.21,80.17 JP6.4
ARDUKOM/D4
  Top 0.61: 18.26,78.58 19.84,78.58 20.22,78.96 MCU3.2
  Top 0.813: JP6.5 7.62,77.63 8.57,78.58 18.26,78.58
ARDUKOM/D5
  Top 0.61: U5.4 29.32,79.22 28.42,79.22 26.51,81.12 MCU3.9
ARDUKOM/D6
  Top 0.61: U5.3 U5.2 29.32,81.76 28.42,81.76 28.06,82.11 MCU3.10
ARDUKOM/D7
  Top 0.61: MCU3.11 29.36,82.91 U5.1
ARDUKOM/MISO  (via drill 0.6)
  Top 0.406: MCU3.16 26.95,86.91 | 26.95,88.11 v26.99,88.11
  Top 0.61: 26.95,86.91 26.95,88.11
  Bottom 0.406: 29.37,90.81 29.37,90.8
  Bottom 0.813: JP5.1 29.37,90.8 29.37,88.11 v26.99,88.11
ARDUKOM/MOSI
  Top 0.406: 32.77,87.15 32.61,87 30.32,87
  Top 0.61: MCU3.15 27.37,86.11 28.26,87 30.32,87
  Top 0.813: 32.77,87.15 JP5.4
ARDUKOM/RES  (via drill 0.6)
  Top 0.61: MCU3.29 20.64,83.71 v20.64,83.66
  Bottom 0.61: 26.35,83.98 27.85,83.98 | 26.19,83.98 20.95,83.98 v20.64,83.66
  Bottom 0.813: 26.19,83.98 26.35,83.98 30.8,83.98 31.27,84.45 31.27,85.66 JP5.5
ARDUKOM/SCK
  Top 0.406: 25.08,89.22 25.02,89.15
  Top 0.61: 29.21,89.22 25.08,89.22 | 25.02,89.15 MCU3.17
  Top 0.813: 29.21,89.22 29.21,88.26 JP5.3
BAT+POL
  Top 0.406: BAT3V.+ 63.34,70.01
  Top 0.61: 63.34,70.01 R24.1
  Top 0.813: K12.2 BAT3V.+
  Bottom 0.406: 63.34,70.01 BAT3V.+
  Bottom 0.61: R42.2 63.34,70.01
BZUK/GATE
  Bottom 0.305: 85.25,61.28 85.25,61.44 84.14,61.44 84.14,60.48 84.61,60.48 | 84.61,60.48 85.25,60.48 85.25,60.64 | 85.25,60.64 85.09,60.64 | 85.09,60.64 84.45,60.64 | 84.45,60.64 84.45,60.8 | 85.25,60.64 85.25,61.28 | 85.25,61.28 84.3,61.28 84.3,60.96 | 84.45,60.64 84.3,60.64 84.3,60.96 | 85.09,60.64 85.09,61.12 84.45,61.12 84.45,60.8 | 84.45,60.8 84.93,60.8 84.93,60.96 84.61,60.96 84.61,60.48 | 84.3,60.96 R1.2
  Bottom 0.813: 82.71,60.96 R1.2 | R2.2 82.71,60.96 | 82.71,60.96 T1.3
EXTRAPIN1
  Bottom 0.61: 2.06,92.87 5.56,92.87 5.56,90.49 1.59,90.49 1.59,92.87 2.06,92.87 | 2.06,92.87 2.06,90.65 5.08,90.65 5.08,92.55 2.54,92.55 2.54,90.96 4.6,90.96 4.6,92.23 3.02,92.23 3.02,91.28 4.13,91.28 4.13,91.92 JP9.1 3.81,91.92 3.81,91.6 3.33,91.6
EXTRAPIN2
  Bottom 0.61: 2.06,93.82 5.56,93.82 5.56,96.2 1.59,96.2 1.59,93.82 2.06,93.82 | 2.06,93.82 2.06,95.89 5.24,95.89 5.24,94.14 2.54,94.14 2.54,95.41 4.76,95.41 4.76,94.61 3.02,94.61 | 3.02,94.61 3.02,95.09 4.92,95.09 | 3.02,94.61 3.17,94.46 JP9.2
GND  (via drill 0.6)
  Top 0.406: 56.36,11.43 58.9,11.43 | R8-B.1 67.47,31.75 67.63,31.75 67.79,31.75 | C2.1 67.47,29.84 | R7.1 67.47,26.67 | C1.1 67.47,24.77 | R9.1 67.47,21.59 | C3.1 67.47,19.68 | 67.47,30.16 67.63,30.16 67.79,30.16 | 67.79,26.99 67.63,26.99 67.47,26.99 | 67.79,25.08 67.63,25.08 | 67.63,24.45 67.47,24.45 | 67.47,21.91 67.63,21.91 67.79,21.91 | 67.79,20 67.63,20 67.47,20
  Top 0.61: 83.66,1.91 78.58,1.91 | 67.79,32.07 67.79,31.75 67.79,31.43 | 67.47,29.53 67.47,29.84 67.47,30.16 | 67.47,26.35 67.47,26.67 67.47,26.99 | 67.47,24.45 67.47,24.77 67.47,25.08 | 67.47,21.91 67.47,21.59 67.47,21.27 | 67.47,20 67.47,19.68 67.47,19.37 | 67.63,32.07 67.63,31.75 67.63,31.43 | 67.47,32.07 67.47,31.75 67.47,31.43 | 67.63,30.16 67.63,29.53 | 67.79,30.16 67.79,29.53 | 67.63,26.99 67.63,26.35 | 67.79,26.99 67.79,26.35 | 67.63,25.08 67.63,24.45 | 67.79,25.08 67.79,24.45 | 67.63,21.91 67.63,21.27 | 67.79,21.91 67.79,21.27 | 67.63,20 67.63,19.37 | 67.79,20 67.79,19.37 | R29.1 v48.58,49.85 R41.2
  Top 0.813: MCU1.GND 66.83,33.02 R8-B.1 C2.1 R7.1 C1.1 R9.1 C3.1 66.83,11.43 | K7.1 55.09,10.16 56.36,11.43 | 58.9,11.43 66.83,11.43 | 66.83,11.43 69.06,11.43 69.06,1.91 78.58,1.91 | K5.3 87.47,22.23 v87.47,26.67 | K4A.1 76.04,48.26 94.46,48.26 K9.1 | K6.1 94.46,26.67 v91.92,26.67 91.92,14.61 K2.1 94.46,1.91 83.66,1.91
  Bottom 0.305: 80.01,56.04 80.8,56.04 80.8,59.69
  Bottom 0.406: T1.1 80.8,59.69 | 52.23,35.56 R27.1 | 52.23,51.44 48.58,51.44 R28.1 v48.58,49.85 | K7.1 48.42,10.16 | 50.01,68.1 50.01,54.13 | 45.09,70.17 47.15,68.1
  Bottom 0.61: 50.01,54.13 R28.1 | 48.42,10.16 R37.2 | 47.15,68.1 50.01,68.1 | R40.1 45.09,70.17
  Bottom 0.813: v87.47,26.67 v91.92,26.67 | MCU1.GND 56.99,33.02 54.45,35.56 K1.8 52.23,35.56 52.23,51.44 BAT3V.- 76.04,51.44 K4A.1 76.04,56.52 R2.1 80.49,56.52 T1.1
GND-ED
  Top 0.406: R22.2 82.39,85.72
  Top 0.813: U2.4 82.39,91.12 82.39,85.72 82.39,75.88 86.2,75.88 | 86.2,75.88 K4B.1 | 86.2,75.88 86.2,78.6 U1.4
GND-IZOL  (via drill 0.6)
  Top 0.813: v25.56,12.38 U4.15 32.23,12.38 32.23,14.35 33.66,14.35 | v25.56,4.76 U4.9 | LED1.C 36.35,17.14 JP2.2 | X2.GND 33.66,14.35 | C8.2 33.66,14.35
  Bottom 0.406: 48.42,21.27 JP3.3
  Bottom 0.61: R37.1 48.42,21.27
  Bottom 0.813: 36.04,20.32 42.7,20.32 JP3.3 | 36.04,20.32 36.04,17.14 35.88,17.14 | 35.88,17.14 JP2.2 | v25.56,4.76 v25.56,12.38 25.56,17.78 DC-DC1.5 | 35.88,14.35 X2.GND 38.42,14.35 C9.1 | 35.88,14.35 33.81,14.35 C7.2 | 35.88,17.14 35.88,14.35 | 36.04,20.32 C10.2 C11.2 35.08,22.23 IO1.2
GND-PC  (via drill 0.6)
  Top 0.813: v21.11,12.38 U4.2 15.08,12.38 C5.2 v15.08,13.97 | v21.11,4.76 U4.8
  Bottom 0.813: v21.11,4.76 v21.11,12.38 21.11,17.78 DC-DC1.4 | X1.GND 6.67,11.13 6.67,15.24 10,15.24 | 10,15.24 12.86,15.24 | 12.86,15.24 15.08,15.24 | 15.08,15.24 JP1.2 | 15.08,15.24 v15.08,13.97 | C4.2 12.86,15.24 | C6.2 10,15.24
GND-TP
  Top 0.813: K13.3 60.33,83.19 59.05,83.19 59.05,90.49 U3.4 61.91,90.49 61.91,90.81 67.94,90.81 K14.4
GNDKOM  (via drill 0.6)
  Top 0.406: MCU3.3 21.05,79.79 | 22.54,81.6 22.54,79.82 MCU3.5 | 24.77,81.6 28.57,77.79 29.21,77.79
  Top 0.61: 21.82,81.6 21.05,81.6 21.05,79.79 v21.05,77.46 | 21.82,81.6 22.54,81.6 | MCU3.5 22.62,81.6 24.77,81.6 | MCU3.21 21.82,85.57 | 21.82,85.57 21.82,81.6 | v24.77,86.84 23.5,85.57 21.82,85.57 | v21.05,77.46
  Top 0.813: 28.73,77.79 29.21,77.79 31.34,77.79 31.34,79.17 | 31.34,79.17 31.34,83.19 JP5.6 | 31.34,79.17 U5.5 35.72,79.17 R17.2 | JP6.6 6.83,75.09 9.21,77.47 v21.06,77.47 v21.05,77.46
  Bottom 0.61: 13.65,83.98 18.89,83.98 20.48,85.57 | v21.05,77.46 21.05,77.31 | 21.05,77.31 21.11,77.31 25.08,77.31 25.08,76.59 C14.2 | 21.05,77.31 16.98,77.31 C13.2
  Bottom 0.813: C12.2 v24.77,86.84 24.77,88.74 20.48,88.74 20.48,85.57 | JP5.6 34.92,85.72 40.01,90.81 K16B.2 39.21,90.81 | C15.1 39.21,90.81 | 39.21,90.81 TR1.P$1 | C13.2 | TR2.P$1 TR1.P$1 | TR1.P$1
  Bottom 1.016: 21.11,73.03 21.11,77.31
JP34
  Bottom 0.406: R32.2 JP34.1
  Bottom 0.61: R40.2 R32.2
KOM485-A  (via drill 0.6)
  Top 0.406: 41.12,80.44 K16A.2
  Top 0.813: U5.6 41.12,80.44 | v30.48,93.98 43.81,93.98 43.81,80.64 K16A.2
  Bottom 0.813: K16A.2 40.96,80.49 37.94,80.49 R19.2 R18.2 | TR2.P$2 v30.48,93.98
KOM485-B  (via drill 0.6)
  Top 0.406: R26.2 v49.37,89.69
  Top 0.813: K16B.1 37.62,85.72 37.62,81.71 U5.7 34.29,81.76 | JP4.2 R17.1 | 34.61,81.76 34.29,81.76 | 34.29,81.76 v32.54,81.76
  Bottom 0.406: v49.37,89.69 49.37,93.98 TR1.P$2
  Bottom 0.813: v32.54,81.76 JP4.2 | K16B.1 43.97,85.72 43.97,93.98 TR1.P$2
KOM485-TERM  (via drill 0.6)
  Top 0.406: R34.1 30.32,73.34 30.16,73.34
  Top 0.813: v37.94,76.83 37.94,73.34 30.16,73.34 30,73.34 JP4.1
  Bottom 0.813: R19.1 v37.94,76.83
N$1
  Bottom 0.406: 74.45,21.59 71.44,21.59
  Bottom 0.813: K5.6 79.22,19.68 77.31,21.59 74.45,21.59 | 71.44,21.59 70.64,21.59 R8-A.2
N$2
  Bottom 0.813: C6.1 X1.P$2
N$3
  Top 0.813: U4.7 16.99,6.03 R11.2
N$4
  Top 0.813: U4.6 15.56,7.3 R10.2
N$5
  Bottom 0.813: C9.2 41.75,18.41 X2.SHIELD@1
N$9
  Top 0.813: U4.5 13.65,8.57 13.65,14.92 12.22,14.92 12.22,19.68 JP1.1
  Bottom 0.813: JP1.1 15.08,20.64 19.53,20.64 R12.1
N$10  (via drill 0.6)
  Top 0.813: JP2.1 R15.1 | U4.13 v30.96,9.84
  Bottom 0.813: v30.96,9.84 R15.1 JP2.1
N$14
  Top 0.813: U4.10 29.69,6.03 30.96,4.76 R14.1
N$15
  Top 0.813: JP3.2 39.53,23.81 38.26,22.54 32.54,22.54 IO1.1
  Bottom 0.813: C11.1 32.54,22.23 IO1.1
N$16
  Top 0.813: U4.11 31.59,7.3 R13.1
N$18
  Top 0.813: LED1.A 36.35,20.64 R16.1
N$21
  Top 0.61: 24.22,77.28 | MCU3.7 24.22,77.28 | 24.22,77.28 24.22,76.04 18.73,76.04 18.73,74.69 Q2.2
  Bottom 0.813: 19.37,76.36 19.37,74.77 | 19.37,74.77 19.37,72.87 | 18.68,74.77 19.37,74.77
  Bottom 1.016: C13.1 18.68,74.76 Q2.2 18.68,74.77
N$22
  Top 0.406: MCU3.8 25.09,79.75
  Top 0.61: Q2.1 25.08,74.69 25.08,79.82 MCU3.8
  Bottom 0.813: 22.86,76.36 22.86,74.77 | 22.86,74.77 22.86,72.87 | 23.5,74.77 22.86,74.77
  Bottom 1.016: C14.1 Q2.1 23.5,74.77
N$28  (via drill 0.6)
  Top 0.61: MCU3.20 22.62,86.84 v22.86,86.84
  Bottom 0.813: v22.86,86.84 C12.1
N$45
  Bottom 0.61: 7.62,86.52 12.22,86.52
N$46
  Bottom 0.61: 7.62,85.25 12.22,85.25
N$47
  Bottom 0.61: 7.62,83.98 12.22,83.98
N$49
  Bottom 0.61: 18.89,86.52 13.65,86.52
N$50
  Bottom 0.61: 18.89,85.25 13.65,85.25
N$51
  Bottom 0.61: 18.89,87.79 13.65,87.79
NAB_9V
  Top 0.813: K8.1 88.11,4.45 88.11,11.43 79.85,11.43 K5.10 79.85,14.55 79.9,14.55 79.9,13.74
NAB_9V-TP
  Top 0.406: 67.94,70.01 K15.5
  Top 0.61: R24.2 67.94,70.01
  Bottom 0.813: K15.5 K13.10
NAPETI_9V  (via drill 0.6)
  Top 0.61: D1.A 90.65,35.56
  Top 0.813: K8.3 91.44,11.91 90.65,12.7 90.65,33.66 | v92.55,33.66 90.65,33.66 | 90.65,33.66 90.65,35.56
  Bottom 0.813: D2.K 92.55,29.21 v92.55,33.66
OSC1-ED
  Top 0.813: U2.1 83.66,94.93 Q1.2
OSC2-ED
  Top 0.813: U2.2 83.66,93.66 Q1.1
PCD+
  Top 0.813: R11.1 8.89,4.6 8.89,9.21 6.67,9.21 6.67,13.65 8.41,13.65 X1.D+
PCD-
  Top 0.813: R10.1 12.38,6.83 12.38,5.71 10,5.71 10,9.21 12.38,9.21 12.38,13.65 10.39,13.65 X1.D-
PERD+  (via drill 0.6)
  Top 0.813: R14.2 36.67,4.76 v36.67,8.26
  Bottom 0.813: v36.67,8.26 36.67,11.81 X2.D+
PERD-
  Top 0.813: R13.2 35.08,6.99 35.08,12.06 36.67,12.06 36.67,9.84 38.96,9.84 X2.D-
PIEZOMINUS
  Bottom 0.406: R23.1 88.58,65.48
  Bottom 0.813: T1.2 80.49,65.48 88.58,65.48 90.65,65.48 BUZZ.-
PIEZOPLUS
  Bottom 0.813: R3.2 94.46,57.71 BUZZ.+
PLUS_9V
  Bottom 0.61: 83.66,1.91 78.58,1.91
  Bottom 0.813: K8.2 89.38,6.99 89.38,1.91 83.66,1.91 | 78.58,1.91 53.18,1.91 K7.2
TEP-CRIT-TP
  Top 0.813: K14.2 65.41,89.22 U3.3
TEP-INT-TP  (via drill 0.6)
  Top 0.406: 53.66,82.87 53.66,83.19 R26.1 v49.37,79.85
  Top 0.813: U3.5 53.66,90.49 53.66,82.87 53.66,73.34 K15.1
  Bottom 0.406: R31.1 v49.37,79.85
TINY/B0
  Top 0.61: 30.51,61.94 JP27.1
  Top 0.813: SJ-B0.2 30.51,61.94
TINY/B1
  Top 0.813: SJ-B1.2 30.51,59.4 JP28.1
TINY/B2
  Top 0.813: SJ-B2.2 30.51,54.26 JP29.1
TINY/B3  (via drill 0.6)
  Top 0.61: 43.15,50.93 43.18,50.96
  Top 0.813: 43.18,50.96 43.21,50.96 R20.1 | 45.88,54.61 MCU2.2 40.96,54.61 v40.96,50.96 43.15,50.96 43.15,50.93
  Bottom 0.813: v40.96,50.96 40.96,44.93 JP31.1
TINY/B4  (via drill 0.6)
  Top 0.61: 38.89,50.96 38.89,50.93 R21.1
  Top 0.813: 38.35,50.96 38.89,50.96 v39.69,50.96 39.69,55.88 MCU2.3 45.88,55.88
  Bottom 0.813: v39.69,50.96 39.69,47.31 36.35,47.31 JP32.1
TINY/B5
  Top 0.813: SJ-B5.2 30.51,51.78 JP30.1
TINY/CAN1
  Bottom 0.813: CAN1.1 9.14,41.59 JP18.1
TINY/CAN2
  Bottom 0.61: 8,47.37 10.29,47.37
  Bottom 0.813: JP19.1 13.21,46.67 12.51,47.37 10.29,47.37 | CAN1.2 8,47.37
TINY/CAN3
  Bottom 0.61: 8,50.23 10.41,50.23
  Bottom 0.813: JP20.1 13.21,51.75 11.68,50.23 10.41,50.23 | CAN1.3 8,50.23
TINY/CAN4
  Bottom 0.61: 8,53.09 9.97,53.09
  Bottom 0.813: 9.97,53.09 13.72,56.83 JP21.1 | CAN1.4 8,53.09
TINY/CAN5
  Bottom 0.406: 15.24,68.1 JP22.1
  Bottom 0.61: R30.2 15.24,68.1
  Bottom 0.813: CAN1.5 12.19,61.91 JP22.1
TINY/CAN6
  Bottom 0.813: CAN1.6 11.65,45.94 13.46,44.13 JP23.1
TINY/CAN7
  Bottom 0.813: CAN1.7 12.54,48.8 12.95,49.21 JP24.1
TINY/CAN8
  Bottom 0.813: CAN1.8 10.57,51.66 13.21,54.29 JP25.1
TINY/CAN9
  Bottom 0.813: CAN1.9 13.94,59.37 JP26.1
TINY/GND  (via drill 0.6)
  Top 0.406: JP94.1 44.77,69.22 R35.1 45.24,70.01 47.15,68.1 | JP93.1 R39.1 | v51.44,70.01 49.53,68.1
  Top 0.61: 42.86,57.15 43.34,57.15 | R29.2 v48.58,39.37 | R41.1 48.58,68.1 | 48.58,68.1 48.1,68.1 47.15,68.1 | 49.53,68.1 48.58,68.1
  Top 0.813: MCU2.4 42.86,57.15 45.47,57.15 | 45.47,57.15 45.47,63.12 43.34,63.12 43.31,63.15 JP10.6 | 43.34,57.15 v43.34,58.58 | 45.47,57.15 45.88,57.15
  Bottom 0.406: R27.2 46.99,35.24 45.4,35.24 | R28.2 48.58,63.15 JP10.6
  Bottom 0.61: v48.58,39.37 48.58,35.56 R27.2 | R42.1 v51.44,70.01
  Bottom 0.813: C16.2 43.02,65.72 | 43.02,65.72 JP10.6 | JP94.1 44.77,65.72 43.02,65.72 | v43.34,58.58 43.34,46.83 45.4,46.83 45.4,35.24 45.4,33.97 JP100.1 JP99.1 JP98.1 JP97.1 JP93.1
TINY/MISO/PB1  (via drill 0.6)
  Top 0.61: 37.08,55.82 36.89,56.01 | 38.37,55.82 37.96,55.82 MCU2.6
  Top 0.813: 38.37,55.82 37.08,55.82 | 34.54,59.37 34.54,58.36 v36.01,56.9 36.89,56.01 | 34.54,59.37 34.54,59.44 | SJ-B1.1 34.51,59.4 34.54,59.37
  Bottom 0.813: v36.01,56.9 36.01,60.61 JP10.1
TINY/MOSI/PB0
  Top 0.61: 37.47,57.47 37.78,57.15 MCU2.5
  Top 0.813: 35.42,61.91 35.42,64.71 40.48,64.71 JP10.4 | 35.42,61.91 36.01,61.91 36.01,58.9 37.43,57.47 37.47,57.47 | 35.42,61.91 34.45,61.91 SJ-B0.1
TINY/RES/PB5  (via drill 0.6)
  Top 0.61: 45.47,53.34 v45.47,51.85
  Top 0.813: SJ-B5.1 34.42,46.93 45.4,46.93 45.4,53.34 | 45.4,53.34 42.93,53.34 MCU2.1 | 45.4,53.34 45.47,53.34 45.88,53.34
  Bottom 0.813: v45.47,51.85 45.47,60.61 JP10.5
TINY/SCK/PB2  (via drill 0.6)
  Top 0.61: 38.44,54.67 37.96,54.67 MCU2.7
  Top 0.813: 38.44,54.67 v36.04,54.67 34.58,54.67 34.58,54.42 SJ-B2.1 34.42,54.61 34.61,54.61
  Bottom 0.813: JP10.3 40.48,54.67 v36.04,54.67
TINY/SOIC1
  Top 0.813: EMPTY1.1 41.27,38.42 41.27,36.51 | 41.26,36.51 41.27,36.51 | 41.27,36.51 JP14.1
  Bottom 0.406: EMPTY2.8 40.39,39.31 41.27,38.42
  Bottom 0.813: 41.27,38.42 41.27,36.51 JP14.1
TINY/SOIC2
  Top 0.813: EMPTY1.2 42.55,39.69 JP15.1
  Bottom 0.406: EMPTY2.7 41.34,39.94 42.23,39.05
  Bottom 0.813: 42.23,39.05 JP15.1
TINY/SOIC3
  Top 0.813: EMPTY1.3 42.55,40.96 JP16.1
  Bottom 0.406: EMPTY2.6 41.21,40.58 42.23,41.59
  Bottom 0.813: 42.23,41.59 JP16.1
TINY/SOIC4
  Top 0.813: EMPTY1.4 41.27,42.23 41.27,44.13 | 41.27,44.13 41.26,44.13 | 41.27,44.13 JP17.1
  Bottom 0.406: EMPTY2.5 40.26,41.21 40.96,41.91
  Bottom 0.813: 40.96,41.91 40.96,43.5 43.18,43.5 JP17.1
TINY/SOIC5
  Top 0.813: JP13.1 32.54,44.13 32.54,42.23 EMPTY1.5
  Bottom 0.406: EMPTY2.4 33.08,41.21 32.38,41.91
  Bottom 0.813: 32.38,41.91 32.38,44.13 JP13.1
TINY/SOIC6
  Top 0.813: EMPTY1.6 31.11,40.96 JP12.1
  Bottom 0.406: EMPTY2.3 32.45,40.58 31.43,41.59
  Bottom 0.813: 31.43,41.59 JP12.1
TINY/SOIC7
  Top 0.813: EMPTY1.7 31.11,39.69 JP11.1
  Bottom 0.406: EMPTY2.2 32.32,39.94 31.43,39.05
  Bottom 0.813: 31.43,39.05 JP11.1
TINY/SOIC8
  Top 0.813: EMPTY1.8 32.54,38.42 32.54,36.51 JP108.1
  Bottom 0.406: EMPTY2.1 33.27,39.31 32.38,38.42
  Bottom 0.813: 32.38,38.42 32.38,36.51 JP108.1
TINY/VCC  (via drill 0.6)
  Top 0.406: 36.83,69.06 JP95.1 | JP104.1 15.4,33.97 R38.1
  Top 0.61: MCU2.8 38.67,53.34 | R34.2 36.83,69.06
  Top 0.813: R20.2 R21.2 38.35,49.02 38.35,48.96 v36.35,48.96 36.35,53.34 MCU2.8 | JP104.1 JP101.1 JP103.1 JP106.1 JP105.1
  Bottom 0.813: 34.38,63.15 JP10.2 37.94,65.72 | 34.38,63.15 34.38,48.96 v36.35,48.96 | 37.94,65.72 C16.1 | JP95.1 36.83,65.72 37.94,65.72 | JP105.1 31.59,33.97 33.97,36.35 36.83,36.35 36.83,43.02 34.29,43.02 34.29,63.15 34.38,63.15
VBUS-PC  (via drill 0.6)
  Top 0.406: 19.58,30.48 DC-DC1.1
  Top 0.61: R38.2 19.58,30.48
  Top 0.813: U4.1 18.89,13.65 18.89,16.03 v19.53,16.03 21.75,16.03 21.75,25.4 19.58,25.4 DC-DC1.1
  Bottom 0.813: 19.58,25.4 DC-DC1.1 | X1.VBUS 12.86,11.13 C4.1 18.89,12.06 18.89,16.03 v19.53,16.03
  Bottom 1.016: DC-DC1.1 19.53,25.4 R12.2
VBUS-PER  (via drill 0.6)
  Top 0.406: R36.1 47.78,26.35 | 47.78,26.35 48.42,26.35 | 47.78,26.35 JP3.1 43.66,30.32
  Top 0.61: R39.2 43.66,30.32
  Top 0.813: U4.16 27.94,15.88 24.92,15.88 24.92,22.86 DC-DC1.7 | DC-DC1.7 27.15,21.59 R15.2 | DC-DC1.7 27.15,27.62 37.62,27.62 IO1.3 | R16.2 v40.16,22.23
  Bottom 0.813: X2.VBUS 38.96,6.03 34.13,6.03 | 34.13,6.03 29.37,6.03 29.37,22.86 DC-DC1.7 | C7.1 34.13,12.06 34.13,6.03 | JP3.1 37.62,26.35 IO1.3 37.62,22.23 C10.1 v40.16,22.23
VCCKOM  (via drill 0.6)
  Top 0.406: 36.2,83.14 v36.2,83.19 | 34.29,83.03 U5.8 | 27.94,90.01 27.94,90.17 | R35.2 41.27,69.22 41.27,74.93 41.12,74.93 K16A.1
  Top 0.61: MCU3.6 23.42,78.37 v22.61,78.37 21.82,78.37 MCU3.4 | MCU3.18 24.22,89.47 24.77,90.01 27.94,90.01 | 36.2,82.98 v36.2,83.19
  Top 0.813: 36.2,83.03 v36.2,83.19 36.2,90.8 JP5.2 33.66,90.8 33.66,92.71 27.94,92.71 JP8.9 27.94,90.17 | U5.8 36.2,82.98
  Bottom 0.406: 22.61,78.48 v22.61,78.37 | R31.2 49.37,72.07 41.27,72.07 41.27,75.56 K16A.1
  Bottom 0.61: 22.51,78.42 22.61,78.42 v22.61,78.37 | 7.62,87.79 10.16,87.79 12.22,87.79
  Bottom 0.813: 22.51,78.42 27.3,78.42 | 27.3,78.42 30.8,78.42 30.8,81.92 31.91,83.03 36.04,83.03 v36.2,83.19 R18.1 | 27.3,78.42 27.3,73.34 34.77,73.34 34.77,75.56 K16A.1 | 10.16,87.79 10.16,89.85 27.94,89.85 JP8.9 | C15.2 33.72,90.81 33.72,90.8 JP5.2
VDD1
  Top 0.813: U4.3 U4.4 15.08,9.84 C5.1
VDD2
  Top 0.813: U4.12 33.66,8.57 33.66,11.11 | 33.66,11.11 U4.14 | C8.1 33.66,11.11
(copper drawn outside any net)
  shapes: Bottom circle x4, Top circle x4

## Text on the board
tPlace: A5 | A4 | A3 | A2 | A1 | A0 | A7 | A6 | +5V | 1 | ISP | RTC | 6 | T-CR | GND | J-Y | GND | LM92 | D0 | B0 | D1 | B | ATMega / KOM:485 | U1 | SDA | J-X | D2 | D3 | A | SRAM | D4 | B2 | B1 | 4 | SCL | U2 | BZK | NAB | +5V | +5V | T-INT | GND | Term. | 1 | +5V | ISP | GND | +3V | PB0 | 4 | D | G | - | 1 | + | BUZZ | PB1 | S | PB2 | 1 | 6 | PB5 | GND | PB4 | PB3 | RST | Tx | Rx | 12V | 8 | Schott. | Vcc | GND | C | GND | R | U2 | USB izolator | UB | 5V | C | R | + | 9V | X | C | U1 | R | B | GND | SP-U | Y | SP-D | Arduino Nano | Joystick | 1 | G | GND | ON | BAT | OFF | +9V / BAT
bPlace: A5 | A4 | A3 | A2 | A1 | A0 | A7 | A6 | +5V | GND | RTC + SRAM | 6 | +5V | D0 | B0 | B | D1 | D2 | GND | A | D3 | B2 | B1 | D4 | GND | +5V | 4 | 1 | +3V | 4 | D | 5 | 3V-OFF | G | 9 | 5 | S | 9 | 4 | 8 | GND | 1 | 6 | 3 | RST | 7 | hodiny | Astronomicke | 2 | Tx | Ver: 4.7 | 6 | 1 | 6 | Rx | 1 | 12V | 8 | GND | Vcc | GND | 5V6 | hodiny.astromik.org | SDA | +5V | Joystick | + | SCL | GND | X | U2 | U1 | B | BZK | J-X | Y | 1 | NAB | J-Y | G | Perif. | GND | PC | ON | BAT | OFF | +9V / BAT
